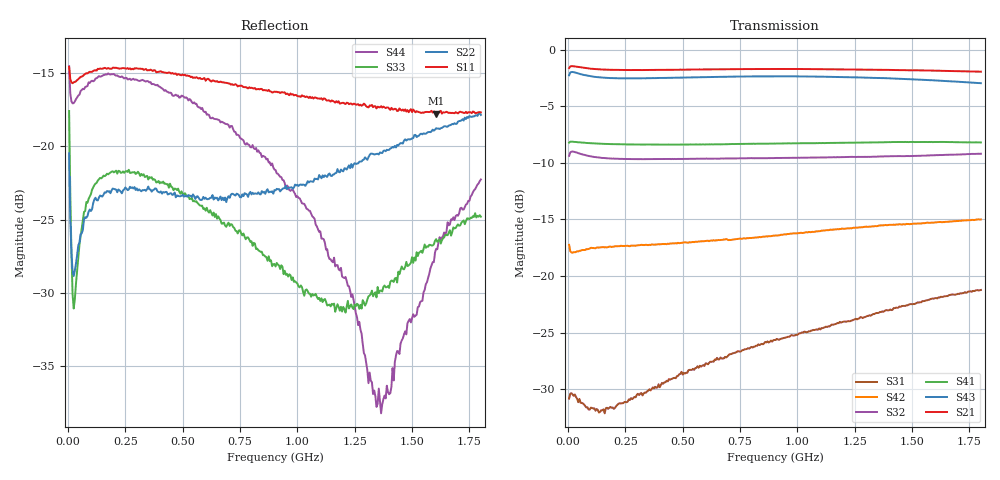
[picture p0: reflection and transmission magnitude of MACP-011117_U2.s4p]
!Agilent Technologies,E5071C,MY46630996,B.13.30
!Date: Tue Jan 23 09:26:42 2024
!Data & Calibration Information:
!MACP-011117 soldered onto PT-0013779 with F connectors, Calibration PT-0003645-TRL. Port1 (pin1) Port2 (pin5) Port3 (pin4) Port4 (pin3)
!Freq	S11:SOLT4(ON)	S12:SOLT4(ON)	S13:SOLT4(ON)	S14:SOLT4(ON)
!	S21:SOLT4(ON)	S22:SOLT4(ON)	S23:SOLT4(ON)	S24:SOLT4(ON)
!	S31:SOLT4(ON)	S32:SOLT4(ON)	S33:SOLT4(ON)	S34:SOLT4(ON)
!	S41:SOLT4(ON)	S42:SOLT4(ON)	S43:SOLT4(ON)	S44:SOLT4(ON)
!PortZ  Port1:75+j0  Port2:75+j0  Port3:75+j0  Port4:75+j0
!Above PortZ is port z conversion or system Z0 setting when saving the data.
!When reading, reference impedance value at option line is always used.
# Hz S MA R 75
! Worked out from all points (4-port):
!   360 points, 5 MHz to 1.8 GHz, reference 75 ohm
!   strongest paths, dB at 5 MHz, 455 MHz, 905 MHz, 1.355 GHz, 1.8 GHz:
!     S21: -1.6, -1.8, -1.7, -1.8, -1.9
!     S43: -2.3, -2.5, -2.4, -2.5, -3.0
!     S41: -8.2, -8.4, -8.3, -8.2, -8.2
!     S32: -9.4, -9.7, -9.6, -9.4, -9.2
!     S42: -17.2, -17.1, -16.4, -15.5, -15.0
!     S31: -30.8, -29.1, -25.6, -23.2, -21.2
!   lowest |S11| = -17.8 dB at 1.605 GHz (marker M1), VSWR 1.30, Z = 58.4 + j4.57 ohm
!   |S11| at or under -10 dB: start of sweep to end of sweep
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5000000  0.1862 163.6  0.83 3.6  0.02977 32.4  0.3915 -178.6
         0.8295 3.9  0.0945 130.4  0.337 8.8  0.1352 173.5
         0.02878 32.1  0.3397 9.1  0.1317 119.3  0.771 6.3
         0.3887 -178.5  0.1374 173.4  0.771 6.4  0.1873 155.1
2.5e7  0.165 178.7  0.8446 -0.3  0.02974 3.9  0.3918 178.4
       0.8439 -0.3  0.03612 173.4  0.3545 0.5  0.1272 178.1
       0.02956 3.4  0.3542 0.4  0.028 165.7  0.7951 -0.5
       0.3915 178.4  0.1277 178.2  0.7955 -0.5  0.1402 177.1
1.95e8  0.185 178.4  0.8142 -3.9  0.02634 12.0  0.3826 167.9
        0.8148 -3.9  0.07173 -165.8  0.3303 -2.8  0.1349 171.7
        0.02627 13.4  0.3301 -2.7  0.08213 -171.1  0.7488 -6.6
        0.3828 167.9  0.1348 171.6  0.7488 -6.6  0.1759 171.5
8.9e8  0.1523 164.5  0.8213 -15.1  0.04837 23.1  0.3836 128.8
       0.8219 -15.1  0.07019 -148.0  0.3323 -6.5  0.1521 138.3
       0.05134 24.3  0.3319 -6.5  0.03901 175.0  0.762 -26.9
       0.3845 128.9  0.1503 137.4  0.762 -26.9  0.08736 123.3
1.365e9  0.1368 162.3  0.8136 -24.0  0.06411 13.6  0.3876 102.3
         0.8149 -24.0  0.09494 -132.2  0.3377 -10.2  0.1691 114.0
         0.06935 14.9  0.3377 -10.2  0.03225 -129.3  0.749 -44.0
         0.3897 102.6  0.1675 112.8  0.7492 -44.0  0.01231 149.2
1.605e9  0.1291 162.7  0.8052 -28.4  0.07401 5.7  0.3879 89.1
         0.8074 -28.6  0.1151 -132.1  0.3424 -12.4  0.1757 102.2
         0.07991 6.7  0.3423 -12.3  0.04823 -118.0  0.7312 -53.2
         0.391 89.1  0.1726 100.9  0.7309 -53.2  0.04472 -137.8
1.8e9  0.1304 163.7  0.7987 -32.0  0.08063 -2.5  0.3871 78.3
       0.7995 -32.2  0.1278 -130.1  0.3464 -14.5  0.1809 92.9
       0.08682 -2.0  0.347 -14.4  0.05752 -114.5  0.7105 -60.9
       0.3892 78.3  0.1779 91.6  0.7111 -60.9  0.07702 -137.3
